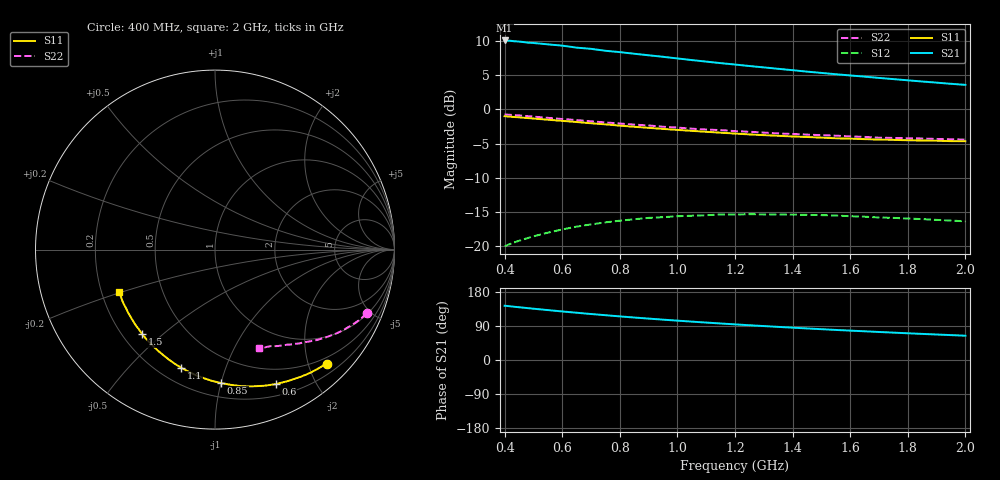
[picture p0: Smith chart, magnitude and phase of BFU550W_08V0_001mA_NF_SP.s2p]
! Filename:  P:\Prog\Test\Noise\ATS_data\Testdata_Net\06 Compressed Noise after Statistics\BFU550W_APM2013_11_D05_08p0V_001mA_NF_CM01_D.sf
! Date/Time: Tue 26/Mar/2013 16:25:22
! BFU550W_APM2013_11_D05_08p0V_1to35mA_NF_CM01_Bias1_R.sf
! Noise Parameter Data File
! BFU550W_APM2013_11_D05_08p0V_1to35mA_NF_CM01
! Date/time: Mon Mar 25 14:39:45 2013
! freq range =  0.4000 to  2.0000 GHz, 37 points
! bias range =  0.9950 to 34.9900 mA, 9 points
! bias supplies used: 1 1 0 0 0 0
! VAR bias_mode= 1  ! Specify V_out, I_out
! VAR bias_var = 1  ! Bias variable = I_out
! VAR V_out= 8.000000
! VAR I_out= 0.995000
! VAR V_in= 0.774100
! VAR I_in= 0.009700
! Device data file deembeded for feedlines and parallel
! Original file: \06 Compressed Noise after Statistics\BFU550W_APM2013_11_D05_08p0V_001mA_NF_CM01_R.sf
! Feed-files: PR019V01_070313_Feed1.s2p, PR019V01_070313_Feed2.s2p
! Parallel-file: PR019V01_070313_Par.s2p
# MHz S MA R 50
!  Freq-MHz  S11-mag  S11-arg  S21-mag  S21-arg  S12-mag  S12-arg  S22-mag  S22-arg
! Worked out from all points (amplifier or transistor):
!   37 points, 400 MHz to 2 GHz, reference 50 ohm
!   highest |S21| = 10.0 dB at 400 MHz (marker M1)
!   |S21| within 3 dB of that: start of sweep to 1.082 GHz
!   unconditionally stable (mu >= 1): nowhere
!   at 500 MHz: K = 0.20, MSG = 14.1 dB, |S12| = -18.5 dB
!   at 1.1 GHz: K = 0.42, MSG = 11.2 dB, |S12| = -15.4 dB
!   at 2 GHz: K = 0.81, MSG = 9.9 dB, |S12| = -16.3 dB
!   lowest NFmin = 0.47 dB at 420 MHz
!   S11 on the Smith chart (normalised r, x): 400 MHz: 0.39, -2.32; 600 MHz: 0.32, -1.50; 850 MHz: 0.30, -1.00; 1.1 GHz: 0.29, -0.71; 1.5 GHz: 0.28, -0.43; 2 GHz: 0.27, -0.20
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400  0.8885 -45.6  3.166 143.3  0.1005 61.7  0.916 -22.8
420  0.8814 -47.8  3.149 141.6  0.1045 60.5  0.9099 -23.8
460  0.8688 -51.9  3.093 138.5  0.1118 58.2  0.8971 -25.6
480  0.8619 -53.8  3.051 136.9  0.1152 57.0  0.8901 -26.6
500  0.8548 -56.0  3.035 135.4  0.1185 55.9  0.8831 -27.4
600  0.8221 -65.8  2.903 128.1  0.1331 50.8  0.8481 -31.5
650  0.8065 -70.2  2.808 124.8  0.1395 48.5  0.8333 -33.3
700  0.7895 -74.8  2.751 121.3  0.1448 46.1  0.8161 -35.3
750  0.7752 -79.0  2.664 118.2  0.1499 44.1  0.8013 -36.8
800  0.7589 -83.3  2.603 115.1  0.1541 42.1  0.7862 -38.5
850  0.7443 -87.4  2.534 112.1  0.1579 40.2  0.772 -40.0
950  0.7182 -95.2  2.407 106.5  0.1635 36.8  0.745 -43.0
1000  0.7064 -99.0  2.341 103.8  0.1661 35.2  0.7345 -44.2
1100  0.6844 -106.0  2.221 98.8  0.169 32.5  0.7106 -46.8
1200  0.6646 -112.8  2.115 94.0  0.1709 30.0  0.6921 -49.3
1250  0.6549 -116.0  2.062 91.7  0.1719 28.9  0.6853 -50.2
1350  0.6401 -122.2  1.968 87.4  0.171 27.1  0.666 -52.6
1500  0.6209 -131.0  1.837 81.3  0.1692 24.8  0.647 -55.8
1600  0.6103 -136.6  1.76 77.5  0.1662 23.8  0.6338 -58.1
1750  0.5979 -144.2  1.656 72.2  0.1616 23.2  0.6177 -61.0
1850  0.5918 -149.1  1.591 68.9  0.1583 23.1  0.6116 -63.1
2000  0.5842 -156.2  1.504 64.1  0.1525 24.0  0.5997 -66.2
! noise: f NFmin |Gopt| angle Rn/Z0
400  0.4854  0.6554  31.16  0.3041
460  0.5083  0.6614  35.59  0.3176
600  0.6269  0.6325  43.06  0.3187
800  0.6412  0.6333  60.18  0.2631
1000  0.8022  0.6487  70.67  0.2883
1200  0.8015  0.6625  87.2  0.2313
1400  0.8486  0.6132  101.3  0.1868
1600  0.7734  0.5612  118.1  0.1294
1800  1.006  0.6135  126  0.1263
2000  1.082  0.625  141.1  0.0918
